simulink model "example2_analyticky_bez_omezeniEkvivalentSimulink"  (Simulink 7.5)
settings: Solver=ode45  StartTime=0.0  StopTime=10000  RelTol=1e-3
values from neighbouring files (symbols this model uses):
  A = [0 0.0001 0;0 0 0.0001;-2.4 -0.25 -0.005]    [example_3_7_1_podklad.m]    (also in example_3_7_2_podklad.m; example_3_7_3_podklad.m)
  B = [0;0;3]    [example_3_7_1_podklad.m]    (also in example_3_7_2_podklad.m; example_3_7_3_podklad.m)
  C = [1 0 0]    [example_3_7_1_podklad.m]    (also in example_3_7_2_podklad.m; example_3_7_3_podklad.m)
  D = 0    [example_3_7_1_podklad.m]    (also in example_3_7_2_podklad.m; example_3_7_3_podklad.m)
  Kr = sum(G(1,:))    [example_3_7_1_podklad.m]
  Kx = F(1,:)    [example_3_7_1_podklad.m]
  Ts = 100    [example_3_7_1_podklad.m]    (also in example_3_7_2_podklad.m; example_3_7_3_podklad.m)
undefined symbols (not defined in the file or in its folder): sigbuilder_block
libraries: simulink x1

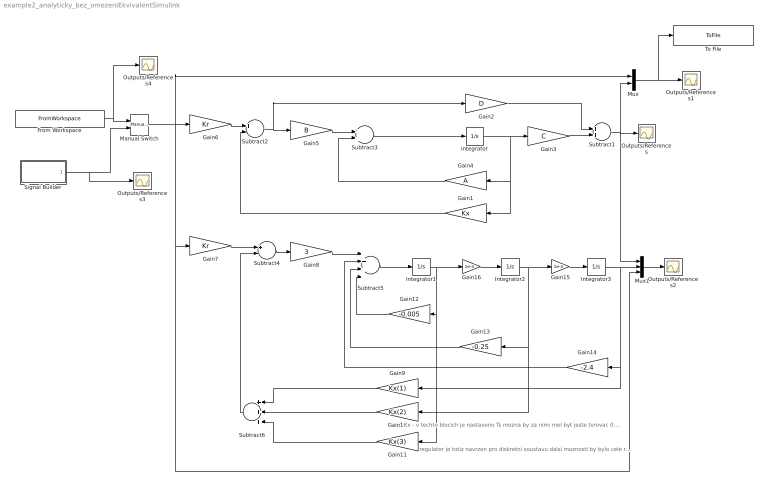
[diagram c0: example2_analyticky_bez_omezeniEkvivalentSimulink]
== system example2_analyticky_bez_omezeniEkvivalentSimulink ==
  note: Kx - v techto blocich je nastaveno Ts mozna by za nimi mel byt jeste tvrovac 0.radu
  note: regulator je totiz navrzen pro diskretni soustavu dalsi moznosti by bylo cele regul. schema predelat na diskretni
  From Workspace : FromWorkspace  VariableName=[100*((0:length(Ref)-1))' Ref']  SampleTime=100  OutputAfterFinalValue=Holding final value
  Gain1 : Gain  Gain=Kx  Multiplication=Matrix(K*u)  ParameterDataType=fixdt(1, 16)  ParameterScaling=2^0  OutDataType=fixdt(1, 16)  OutScaling=2^0  SampleTime=Ts
  Gain10 : Gain  Gain=Kx(2)  ParameterDataType=fixdt(1, 16)  ParameterScaling=2^0  OutDataType=fixdt(1, 16)  OutScaling=2^0  SampleTime=Ts
  Gain11 : Gain  Gain=Kx(3)  ParameterDataType=fixdt(1, 16)  ParameterScaling=2^0  OutDataType=fixdt(1, 16)  OutScaling=2^0  SampleTime=Ts
  Gain12 : Gain  Gain=-0.005  ParameterDataType=fixdt(1, 16)  ParameterScaling=2^0  OutDataType=fixdt(1, 16)  OutScaling=2^0
  Gain13 : Gain  Gain=-0.25  ParameterDataType=fixdt(1, 16)  ParameterScaling=2^0  OutDataType=fixdt(1, 16)  OutScaling=2^0
  Gain14 : Gain  Gain=-2.4  ParameterDataType=fixdt(1, 16)  ParameterScaling=2^0  OutDataType=fixdt(1, 16)  OutScaling=2^0
  Gain15 : Gain  Gain=1e-4  ParameterDataType=fixdt(1, 16)  ParameterScaling=2^0  OutDataType=fixdt(1, 16)  OutScaling=2^0
  Gain16 : Gain  Gain=1e-4  ParameterDataType=fixdt(1, 16)  ParameterScaling=2^0  OutDataType=fixdt(1, 16)  OutScaling=2^0
  Gain2 : Gain  Gain=D  Multiplication=Matrix(K*u)  ParameterDataType=fixdt(1, 16)  ParameterScaling=2^0  OutDataType=fixdt(1, 16)  OutScaling=2^0
  Gain3 : Gain  Gain=C  Multiplication=Matrix(K*u)  ParameterDataType=fixdt(1, 16)  ParameterScaling=2^0  OutDataType=fixdt(1, 16)  OutScaling=2^0
  Gain4 : Gain  Gain=A  Multiplication=Matrix(K*u)  ParameterDataType=fixdt(1, 16)  ParameterScaling=2^0  OutDataType=fixdt(1, 16)  OutScaling=2^0
  Gain5 : Gain  Gain=B  Multiplication=Matrix(K*u)  ParameterDataType=fixdt(1, 16)  ParameterScaling=2^0  OutDataType=fixdt(1, 16)  OutScaling=2^0
  Gain6 : Gain  Gain=Kr  Multiplication=Matrix(K*u)  ParameterDataType=fixdt(1, 16)  ParameterScaling=2^0  OutDataType=fixdt(1, 16)  OutScaling=2^0
  Gain7 : Gain  Gain=Kr  Multiplication=Matrix(K*u)  ParameterDataType=fixdt(1, 16)  ParameterScaling=2^0  OutDataType=fixdt(1, 16)  OutScaling=2^0
  Gain8 : Gain  Gain=3  ParameterDataType=fixdt(1, 16)  ParameterScaling=2^0  OutDataType=fixdt(1, 16)  OutScaling=2^0
  Gain9 : Gain  Gain=Kx(1)  ParameterDataType=fixdt(1, 16)  ParameterScaling=2^0  OutDataType=fixdt(1, 16)  OutScaling=2^0  SampleTime=Ts
  Integrator{,1..3} (4 alike) : Integrator
  Manual Switch : simulink/Signal Routing/Manual Switch  SystemSampleTime=-1  sw=0  action=0  varsize=off
  Mux : Mux  Inputs=2
  Mux1 : Mux  Inputs=3
  Outputs/References{,1..4} (5 alike) : Scope
  Signal Builder : Subsystem  Tag=STV Subsys  LoadFcn=sigbuilder_block('load');  StartFcn=sigbuilder_block('start');  StopFcn=sigbuilder_block('stop');  ClipboardFcn=sigbuilder_block('clipboard');
  Subtract1 : Sum  OutDataType=fixdt(1, 16)  OutScaling=2^-10
  Subtract2 : Sum  Inputs=+-  OutDataType=fixdt(1, 16)  OutScaling=2^-10
  Subtract3 : Sum  OutDataType=fixdt(1, 16)  OutScaling=2^-10
  Subtract4 : Sum  Inputs=+-  OutDataType=fixdt(1, 16)  OutScaling=2^-10
  Subtract5 : Sum  Inputs=++++  OutDataType=fixdt(1, 16)  OutScaling=2^-10
  Subtract6 : Sum  Inputs=+++  OutDataType=fixdt(1, 16)  OutScaling=2^-10
  To File : ToFile  Filename=simoutStepan  MatrixName=simoutStepan
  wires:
  Integrator/1 -> Gain3/1, Gain4/1, Gain1/1
  Gain3/1 -> Subtract1/2
  Gain2/1 -> Subtract1/1
  Subtract3/1 -> Integrator/1
  Gain4/1 -> Subtract3/2
  Gain5/1 -> Subtract3/1
  Subtract1/1 -> Outputs/References/1, Mux/2, Mux1/1
  Gain6/1 -> Subtract2/1
  Subtract2/1 -> Gain5/1, Gain2/1
  Mux/1 -> Outputs/References1/1, To File/1
  Gain7/1 -> Subtract4/1
  Subtract4/1 -> Gain8/1
  Gain8/1 -> Subtract5/1
  Subtract5/1 -> Integrator1/1
  Integrator1/1 -> Gain12/1, Gain11/1, Gain16/1
  Integrator2/1 -> Gain13/1, Gain10/1, Gain15/1
  Integrator3/1 -> Gain14/1, Gain9/1, Mux1/2
  Gain12/1 -> Subtract5/4
  Gain13/1 -> Subtract5/3
  Gain14/1 -> Subtract5/2
  Gain9/1 -> Subtract6/1
  Gain10/1 -> Subtract6/2
  Gain11/1 -> Subtract6/3
  Subtract6/1 -> Subtract4/2
  Mux1/1 -> Outputs/References2/1
  Gain15/1 -> Integrator3/1
  Gain16/1 -> Integrator2/1
  Gain1/1 -> Subtract2/2
  Manual Switch/1 -> Gain6/1, Mux/1, Gain7/1, Mux1/3
  From Workspace/1 -> Manual Switch/1, Outputs/References4/1
  Signal Builder/1(Signal 2) -> Manual Switch/2, Outputs/References3/1

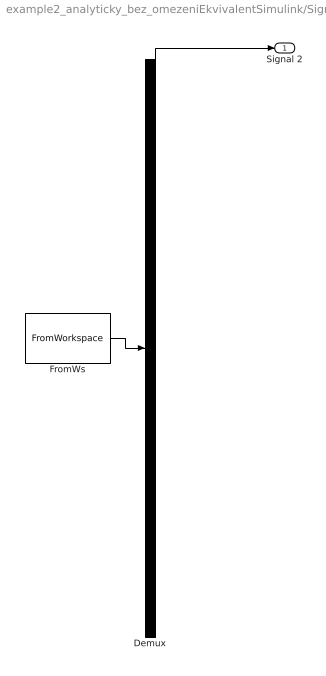
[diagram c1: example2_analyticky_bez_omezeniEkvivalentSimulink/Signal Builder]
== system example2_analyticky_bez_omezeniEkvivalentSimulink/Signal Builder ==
  Demux : Demux  Tag=STV Demux  Outputs=1
  FromWs : FromWorkspace  Tag=STV FromWs  VariableName=tuvar  SampleTime=0  SigBuilderData=DataTag0  VnvData=DataTag1
  Signal 2 : Outport  Tag=STV Outport
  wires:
  FromWs/1 -> Demux/1
  Demux/1 -> Signal 2/1
